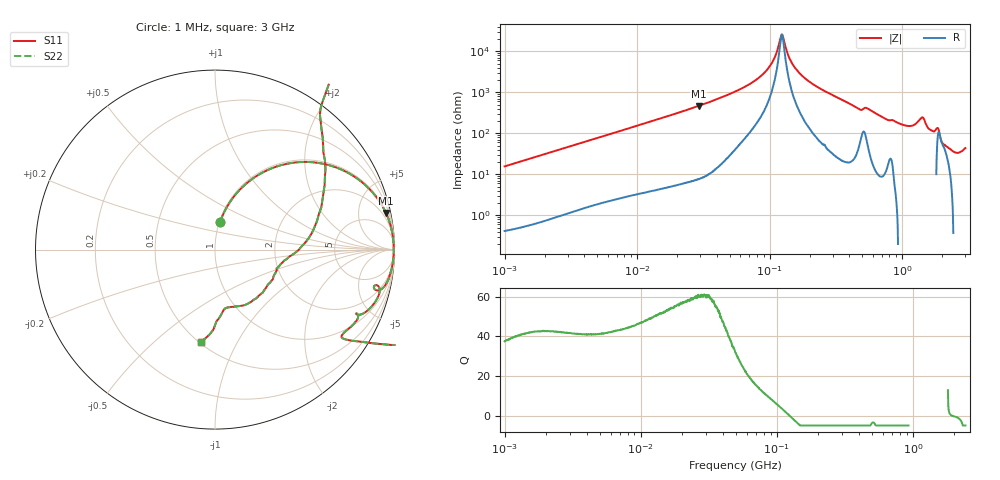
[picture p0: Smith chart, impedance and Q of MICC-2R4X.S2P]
!s-Parameter Generated by FASTRON Sdn. Bhd.
!FASTRON P/N : MICC-2R4X
!Keysight Technologies,E4991B,MY54100416,A.01.15
!Date: Fri Aug 28 09:37:49 2026
!Version  : Rev00 Fri Aug 28 09:37:49 2026
!Data & Calibration Information:
!PortZ  Port1:50+j0  Port2:50+j0
!When reading, reference impedance value at option line is always used.
! Remarks : This data is being provided solely for informational purposes.
!Freq	S11	S21	S12	S22
# Hz S dB R 50
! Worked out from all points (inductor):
!   1601 points, 1 MHz to 3 GHz, reference 50 ohm
!   read as one part in series: L = 2.48 uH near 1.041 MHz
!   highest Q = 60.8 at 29.16 MHz (marker M1), where L = 2.54 uH
!   self-resonance near 123.2 MHz
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1000000  -16.26 79.6  -0.14 -8.8  -0.14 -8.8  -16.26 79.6
3804036  -6.00 58.5  -1.38 -30.1  -1.38 -30.1  -6.00 58.5
1.447069e7  -0.87 24.1  -7.79 -64.8  -7.79 -64.8  -0.87 24.1
2.915663e7  -0.22 12.1  -13.59 -77.0  -13.59 -77.0  -0.22 12.1
5.477226e7  -0.07 5.5  -20.39 -82.3  -20.39 -82.3  -0.07 5.5
9.450168e7  -0.04 1.7  -30.63 -80.5  -30.63 -80.5  -0.04 1.7
1.238204e8  -0.03 -0.0  -48.22 1.2  -48.22 1.2  -0.03 -0.0
1.512587e8  -0.04 -1.3  -33.04 78.6  -33.04 78.6  -0.04 -1.3
2.083556e8  -0.05 -3.5  -24.35 82.8  -24.35 82.8  -0.05 -3.5
7.925923e8  -1.22 -24.6  -7.58 59.9  -7.58 59.9  -1.22 -24.6
1.200675e9  -1.09 -34.6  -4.88 61.3  -4.88 61.3  -1.09 -34.6
1.313842e9  0.23 -30.6  -5.43 77.4  -5.43 77.4  0.23 -30.6
1.395152e9  2.22 -23.5  -5.23 109.6  -5.23 109.6  2.22 -23.5
1.45942e9  4.84 -9.2  -2.20 158.9  -2.20 158.9  4.84 -9.2
1.519029e9  7.83 13.6  3.58 -157.5  3.58 -157.5  7.83 13.6
1.57318e9  8.19 41.6  5.74 -118.3  5.74 -118.3  8.19 41.6
1.613037e9  6.69 52.4  4.81 -100.5  4.81 -100.5  6.69 52.4
1.704314e9  1.32 56.3  0.27 -69.9  0.27 -69.9  1.32 56.3
1.846379e9  -3.61 24.8  -6.25 -34.6  -6.25 -34.6  -3.61 24.8
1.950859e9  -7.38 -4.2  -4.82 3.1  -4.82 3.1  -7.38 -4.2
2.568929e9  -9.64 -78.0  -0.12 19.1  -0.12 19.1  -9.64 -78.0
3e9  -5.66 -98.5  1.54 25.6  1.54 25.6  -5.66 -98.5
